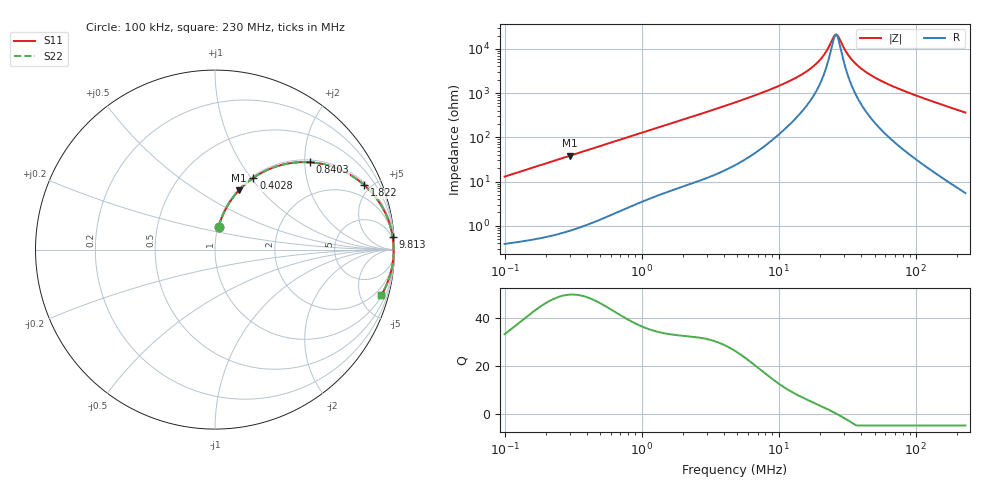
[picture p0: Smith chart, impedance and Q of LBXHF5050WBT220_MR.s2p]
! LBXHF5050WBT220_MR  S-PARAMETER MODEL  ( General Type )
! Model Generated by TAIYO YUDEN Corporation (http://www.ty-top.com)
! Version 1.0
! TAIYO YUDEN Control No. 210719NI43SB-FBB
! Copyright(c) 2021 TAIYO YUDEN CO.,LTD. All Rights Reserved.
! Product Description (link to TY-COMPAS)
! https://ds.yuden.co.jp/TYCOMPAS/or/detail?pn=LBXHF5050WBT220MMR&u=M
! Products Name : Inductors
! Characteristics :
!  Inductance : 22 uH , SRF(min) : 18 MHz , DC Resistance(max) : 0.28 Ohm
!  Rated Current : Saturation :1100 mA , Temp Rise : 800 mA
!  Case Size : 5.0 x 5.0 / 0.197 x 0.197 [mm/inch] , Thickness : 2.2 / 0.087 [mm/inch]
!  (Conditions: Temperature = 25 degC , DC Bias Current/Voltage = 0A / 0V)
! External Node Assignments :
!  1  o---GGG---o  2
! GND o---------o GND
! Frequency Range : 0.1MHz  -  229.966873MHz  [ 402 STEP ]
# MHz S RI R 50
! Freq[MHz].  S11 Real  S11 Imag  S21 Real  S21 Imag  S12 Real  S12 Imag  S22 Real  S22 Imag
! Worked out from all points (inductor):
!   401 points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, 100 kHz to 230 MHz, reference 50 ohm
!   read as one part in series: L = 20.5 uH near 103.9 kHz
!   highest Q = 49.9 at 301.3 kHz (marker M1), where L = 20.4 uH
!   self-resonance near 25.82 MHz
!   S11 on the Smith chart (normalised r, x): 100 kHz: 1.01, +0.26; 402.8 kHz: 1.02, +1.03; 840.3 kHz: 1.06, +2.13; 1.822 MHz: 1.14, +4.57; 9.813 MHz: 3, +28; 230 MHz: 1.11, -7.27
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0.1  0.02 0.1257  0.98 -0.1257  0.98 -0.1257  0.02 0.1257
0.301326  0.1343 0.3311  0.8657 -0.3311  0.8657 -0.3311  0.1343 0.3311
0.365661  0.1842 0.3776  0.8158 -0.3776  0.8158 -0.3776  0.1842 0.3776
0.40281  0.2141 0.4001  0.7859 -0.4001  0.7859 -0.4001  0.2141 0.4001
0.840346  0.5309 0.4863  0.4691 -0.4863  0.4691 -0.4863  0.5309 0.4863
1.337081  0.7333 0.4279  0.2667 -0.4279  0.2667 -0.4279  0.7333 0.4279
1.822319  0.832 0.3589  0.168 -0.3589  0.168 -0.3589  0.832 0.3589
2.843939  0.9204 0.2553  0.0796 -0.2553  0.0796 -0.2553  0.9204 0.2553
4.889189  0.9696 0.1536  0.0304 -0.1536  0.0304 -0.1536  0.9696 0.1536
9.812658  0.9897 0.0693  0.0103 -0.0693  0.0103 -0.0693  0.9897 0.0693
13.9015  0.9928 0.0411  0.00716 -0.0411  0.00716 -0.0411  0.9928 0.0411
17.53523  0.9941 0.0252  0.00588 -0.0252  0.00588 -0.0252  0.9941 0.0252
20.87128  0.9948 0.0141  0.0052 -0.0141  0.0052 -0.0141  0.9948 0.0141
25.3274  0.9953 0.00204  0.00473 -0.00204  0.00473 -0.00204  0.9953 0.00204
26.32686  0.9953 -0.000362  0.00468 0.000362  0.00468 0.000362  0.9953 -0.000362
27.36575  0.9954 -0.00277  0.00464 0.00277  0.00464 0.00277  0.9954 -0.00277
31.94778  0.9954 -0.0125  0.00462 0.0125  0.00462 0.0125  0.9954 -0.0125
37.297  0.9952 -0.0226  0.00485 0.0226  0.00485 0.0226  0.9952 -0.0226
47.04613  0.9943 -0.0388  0.00571 0.0388  0.00571 0.0388  0.9943 -0.0388
64.11956  0.9918 -0.0638  0.0082 0.0638  0.0082 0.0638  0.9918 -0.0638
112.3857  0.9799 -0.1256  0.0201 0.1256  0.0201 0.1256  0.9799 -0.1256
229.9669  0.9264 -0.2536  0.0736 0.2536  0.0736 0.2536  0.9264 -0.2536
